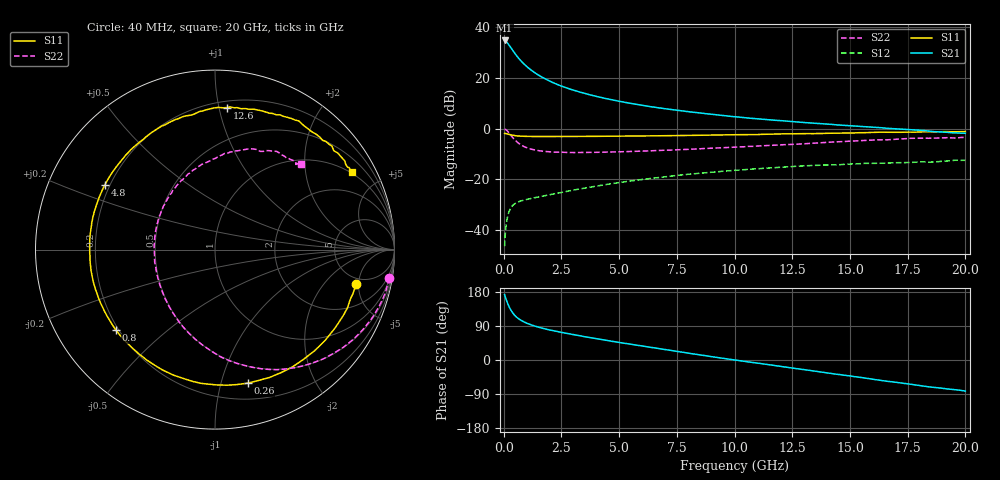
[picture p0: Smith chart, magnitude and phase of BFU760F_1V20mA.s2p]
! Filename:  P:\Prog\Test\Noise\ATS_data\Testdata_Net\Split files Spar\BFU760F_2W_C1_1V_5mA_60mA_Bias5_D.s2p
! Date/Time: Mon 06/Feb/2012 15:06:11
! BFU760_2W_C1_1V_5mA_60mA_Bias5_R.s2p
! MDIF S-parameter v. bias file
! BFU760_2W_C1_1V_5mA_60mA
! Date/time Fri Mar 18 10:56:44 2011
! VAR V_out= 1.0002
! VAR I_out= 19.9700
! VAR V_in= 0.7946
! VAR I_in= 0.0619
! Device data file deembeded for feedlines and parallel
! Original file: \Split files Spar\BFU760_2W_C1_1V_5mA_60mA_Bias5_R.s2p
! Feed-files: PR003V01_101208_Feed1.s2p, PR003V01_101208_Feed2.s2p
! Parallel-file: PR003V01_101208_Par.s2p
# MHz S MA R 50
!  Freq-MHz  S11-mag  S11-arg  S21-mag  S21-arg  S12-mag  S12-arg  S22-mag  S22-arg
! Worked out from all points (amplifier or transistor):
!   167 points, 40 MHz to 20 GHz, reference 50 ohm
!   highest |S21| = 34.9 dB at 40 MHz (marker M1)
!   |S21| within 3 dB of that: start of sweep to 323.2 MHz
!   unconditionally stable (mu >= 1): 4.235 GHz to 15.09 GHz
!   at 550 MHz: K = 0.25, MSG = 29.1 dB, |S12| = -29.3 dB
!   at 4.2 GHz: K = 1.00, MSG = 17.4 dB, |S12| = -22.4 dB
!   at 20 GHz: K = 0.92, MSG = 5.3 dB, |S12| = -12.5 dB
!   S11 on the Smith chart (normalised r, x): 40 MHz: 4.21, -4.69; 260 MHz: 0.34, -1.22; 800 MHz: 0.19, -0.34; 4.8 GHz: 0.18, +0.26; 12.6 GHz: 0.25, +1.06; 20 GHz: 0.96, +3.58
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40  0.8108 -13.6  55.32 172.4  0.004784 83.4  0.9846 -9.3
50  0.8066 -17.8  55.04 169.9  0.006328 84.8  0.9804 -11.9
90  0.8004 -30.2  53.52 162.7  0.01058 76.0  0.9608 -21.5
140  0.7911 -45.4  50.87 154.2  0.01564 68.8  0.9192 -32.9
200  0.7779 -61.9  46.97 145.2  0.02077 61.3  0.8575 -45.2
260  0.766 -76.3  43.05 137.4  0.02473 55.2  0.7932 -56.1
320  0.7544 -89.0  39.36 130.8  0.02779 50.2  0.7321 -65.8
380  0.7449 -99.7  35.94 125.2  0.03011 46.4  0.6769 -74.1
480  0.7316 -113.5  30.86 117.8  0.03299 41.4  0.6042 -86.0
600  0.719 -126.2  26.17 111.0  0.03528 37.8  0.5353 -97.7
800  0.7113 -140.8  20.6 103.0  0.03805 34.4  0.4646 -112.8
1150  0.703 -156.6  14.81 93.5  0.04157 32.9  0.3993 -131.6
1700  0.6998 -171.3  10.2 83.5  0.04678 33.7  0.3589 -150.8
2400  0.6991 176.9  7.236 74.1  0.05394 35.2  0.3431 -166.7
3400  0.7037 164.2  5.134 62.8  0.0658 35.6  0.3396 177.8
4800  0.712 149.6  3.631 48.2  0.08373 33.2  0.3485 161.0
6800  0.7254 131.6  2.553 29.1  0.11 25.7  0.3722 141.5
10200  0.7616 103.8  1.692 -1.6  0.1528 7.5  0.4378 112.7
12600  0.7942 85.1  1.369 -22.0  0.1799 -7.0  0.4919 94.4
13400  0.7982 79.5  1.287 -28.7  0.1882 -12.9  0.5154 88.5
16800  0.8499 53.7  1.004 -57.3  0.2109 -34.3  0.6103 63.8
20000  0.8776 29.4  0.8142 -82.0  0.2375 -55.5  0.6749 44.8
